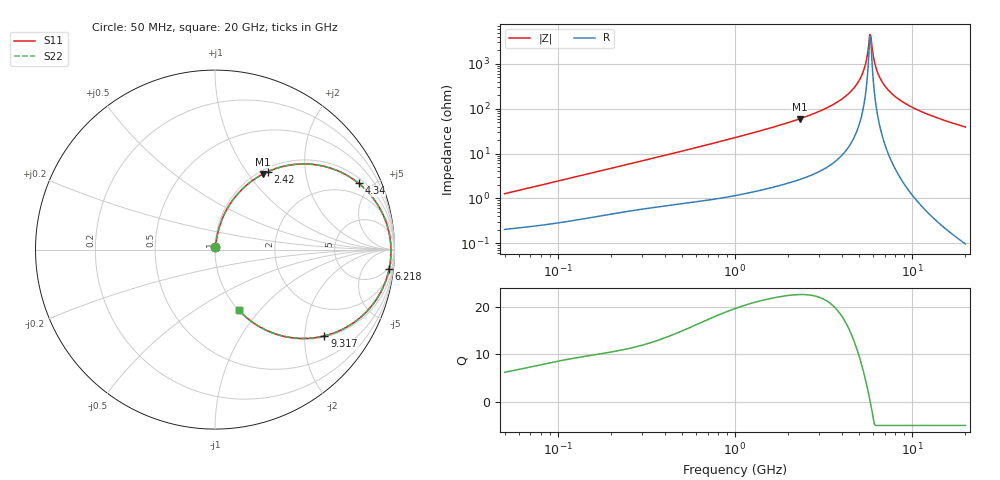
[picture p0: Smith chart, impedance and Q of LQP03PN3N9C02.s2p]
!Murata Part Number: LQP03PN3N9C02
!These Parameters are Measured in Series Mode Connection
!  o--[Z]--o
!Port1  Port2
!  o-------o
!Freq. Start=50[MHz] Stop=20[GHz], 401[Steps]
# Hz S RI R 50
!Freq.(Hz) S11(Real) S11(Imag) S21(Real) S21(Imag) S12(Real) S12(Imag) S22(Real) S22(Imag)
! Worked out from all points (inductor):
!   401 points, 50 MHz to 20 GHz, reference 50 ohm
!   read as one part in series: L = 3.93 nH near 51.52 MHz
!   highest Q = 22.6 at 2.314 GHz (marker M1), where L = 4.07 nH
!   self-resonance near 5.769 GHz
!   S11 on the Smith chart (normalised r, x): 50 MHz: 1.00, +0.03; 2.42 GHz: 1.06, +1.26; 4.34 GHz: 1.27, +4.19; 6.218 GHz: 4, -17; 9.317 GHz: 1.03, -2.51; 20 GHz: 1.00, -0.78
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5e7  0.00218 0.0125  0.9978 -0.0125  0.9978 -0.0125  0.00218 0.0125
1.364002e8  0.00447 0.0322  0.9955 -0.0322  0.9955 -0.0322  0.00447 0.0322
3.721004e8  0.0134 0.0828  0.9866 -0.0828  0.9866 -0.0828  0.0134 0.0828
1e9  0.0584 0.2104  0.9416 -0.2104  0.9416 -0.2104  0.0584 0.2104
1.614971e9  0.1373 0.322  0.8627 -0.322  0.8627 -0.322  0.1373 0.322
2.313601e9  0.269 0.4218  0.731 -0.4218  0.731 -0.4218  0.269 0.4218
2.419936e9  0.2928 0.4334  0.7072 -0.4334  0.7072 -0.4334  0.2928 0.4334
2.728004e9  0.367 0.4602  0.633 -0.4602  0.633 -0.4602  0.367 0.4602
3.519108e9  0.5822 0.4694  0.4178 -0.4694  0.4178 -0.4694  0.5822 0.4694
4.34015e9  0.8002 0.3694  0.1998 -0.3694  0.1998 -0.3694  0.8002 0.3694
4.81993e9  0.8972 0.2638  0.1028 -0.2638  0.1028 -0.2638  0.8972 0.2638
5.194772e9  0.9482 0.1662  0.0518 -0.1662  0.0518 -0.1662  0.9482 0.1662
5.433528e9  0.9682 0.1008  0.0318 -0.1008  0.0318 -0.1008  0.9682 0.1008
5.683258e9  0.9789 0.0323  0.0211 -0.0323  0.0211 -0.0323  0.9789 0.0323
5.769027e9  0.9803 0.00901  0.0197 -0.00901  0.0197 -0.00901  0.9803 0.00901
5.944466e9  0.9797 -0.0376  0.0203 0.0376  0.0203 0.0376  0.9797 -0.0376
6.217679e9  0.9705 -0.1068  0.0295 0.1068  0.0295 0.1068  0.9705 -0.1068
6.701223e9  0.9343 -0.2153  0.0657 0.2153  0.0657 0.2153  0.9343 -0.2153
7.442007e9  0.8487 -0.3412  0.1513 0.3412  0.1513 0.3412  0.8487 -0.3412
9.316812e9  0.6096 -0.481  0.3904 0.481  0.3904 0.481  0.6096 -0.481
1.334722e10  0.3043 -0.4575  0.6957 0.4575  0.6957 0.4575  0.3043 -0.4575
2e10  0.1325 -0.3378  0.8675 0.3378  0.8675 0.3378  0.1325 -0.3378
